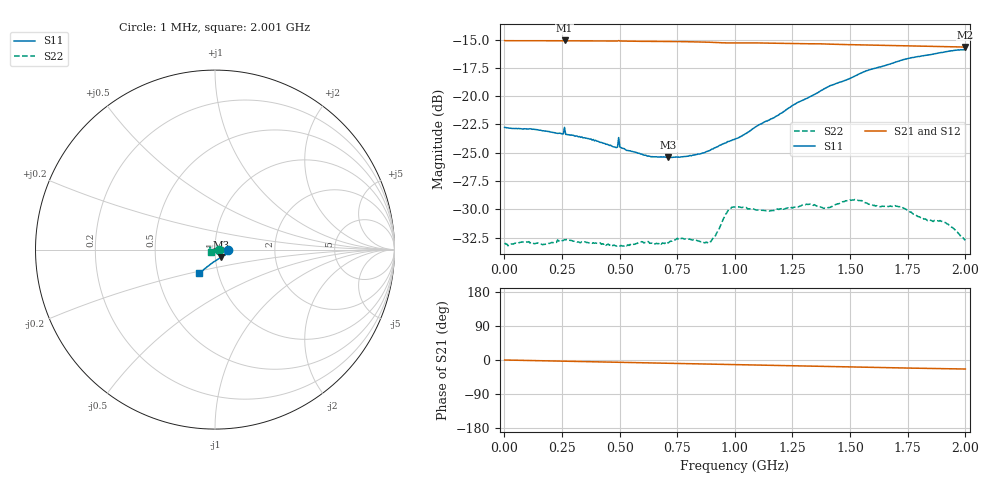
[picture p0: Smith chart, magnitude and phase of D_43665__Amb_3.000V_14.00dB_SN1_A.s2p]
! device id: 43665_
! dir: \\malibu\benchdata\1_engineers\tn_data\43665_75ohm\new\sparar\43665_\amb\3p000v\14p00db
! Serial: 1
! Insertion: A
! Temp: Amb
! VDD: 3.000V
! Attenuation Step: 14.00dB
! IDD: 1.449063e+00mA
! FILE NAME
! DATE 03-27-2009 08:36:48
! CORRECTED  DATA
#  Hz  S  RI  R  75
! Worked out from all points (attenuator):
!   401 points, 1 MHz to 2.001 GHz, reference 75 ohm
!   highest |S21| = -15.08 dB at 261 MHz (marker M1); lowest = -15.7 dB at 2.001 GHz (marker M2)
!   lowest |S11| = -25.4 dB at 711 MHz (marker M3), VSWR 1.11, Z = 79.7 - j6.83 ohm
!   |S11| at or under -10 dB: start of sweep to end of sweep
!   |S22| runs from -33.2 to -29.1 dB; largest |S21 - S12| = 0.00071
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1000000  0.0728 -0.000781  0.1761 -0.000212  0.176 -0.000123  0.0225 -5.4e-05
1.76e8  0.0694 -0.00952  0.1755 -0.00633  0.1756 -0.00642  0.0198 0.01
2.61e8  0.0711 -0.0154  0.1759 -0.00956  0.1753 -0.00952  0.0176 0.0152
3.36e8  0.0635 -0.0186  0.175 -0.0123  0.175 -0.0124  0.0136 0.0182
4.91e8  0.0528 -0.0274  0.1742 -0.0181  0.1742 -0.0182  0.00534 0.0213
5.91e8  0.0436 -0.0344  0.1732 -0.022  0.1733 -0.0219  -0.00185 0.0226
6.71e8  0.0361 -0.04  0.1726 -0.0248  0.1726 -0.0248  -0.00583 0.0216
7.11e8  0.0324 -0.0427  0.1723 -0.0264  0.1723 -0.0263  -0.00784 0.0211
7.76e8  0.0258 -0.0475  0.1715 -0.0289  0.1716 -0.0288  -0.0125 0.0199
8.91e8  0.0127 -0.0561  0.1697 -0.0335  0.1698 -0.0333  -0.0192 0.0125
9.26e8  0.00825 -0.0592  0.1688 -0.0347  0.1689 -0.0345  -0.023 0.0105
9.66e8  0.00431 -0.0625  0.1681 -0.0355  0.1682 -0.0352  -0.0285 0.0112
1.001e9  5.98e-05 -0.0646  0.168 -0.0364  0.1681 -0.0361  -0.03 0.0124
1.156e9  -0.0182 -0.0771  0.1661 -0.042  0.1664 -0.0418  -0.0306 0.00623
1.336e9  -0.0393 -0.0925  0.1633 -0.0481  0.1637 -0.048  -0.033 -0.00337
1.396e9  -0.0465 -0.0983  0.1623 -0.0504  0.1626 -0.0503  -0.0312 -0.00662
1.521e9  -0.0591 -0.1076  0.1597 -0.054  0.1601 -0.054  -0.0331 -0.0113
1.671e9  -0.0718 -0.1184  0.1569 -0.0584  0.1571 -0.0584  -0.0297 -0.0135
1.716e9  -0.0756 -0.1216  0.156 -0.0596  0.1562 -0.0596  -0.0288 -0.0151
1.826e9  -0.0814 -0.1276  0.1539 -0.0624  0.1538 -0.0626  -0.0248 -0.0144
1.911e9  -0.0871 -0.1303  0.1524 -0.0644  0.1525 -0.0643  -0.0238 -0.0142
2.001e9  -0.0899 -0.1325  0.1507 -0.0664  0.1505 -0.0667  -0.0196 -0.0122
